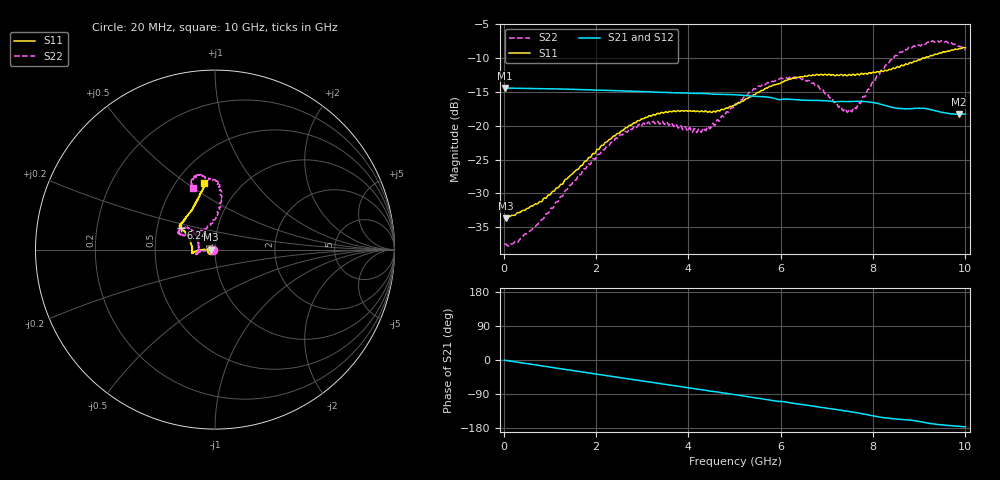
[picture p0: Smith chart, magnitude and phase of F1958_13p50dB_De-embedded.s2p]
! Integrated Device Technology
! Corporate Headquarters
! 6024 Silver Creek Valley Road
! San Jose, CA 95138  USA
! Phone:  1-408-284-8200
! Toll Free:  1-800-223-1366
! Webpage:  http://www.idt.com/
! Timing and RF Division
! 515 Groton Road, Suite 102
! Westford, MA 01886-6024
! Device:  F1958
! Description: 7-bit 0.25 dB Digital Step Attenuator
! Frequency:  0.001 -  6.000 GHz
! Package:  4x4 mm Thin QFN Plastic Package: 24 pin
! Ports:  2 RF, 12 DC
!  Pin  1  = D0
!  Pin  2  = VDD
!  Pin  3  = VMODE
!  Pin  4  = GND
!  Pin  5  = RF1  =  Port 1
!  Pin  6  = GND
!  Pin  7  = GND
!  Pin  8  = GND
!  Pin  9  = GND
!  Pin 10  = GND
!  Pin 11  = GND
!  Pin 12  = GND
!  Pin 13  = GND
!  Pin 14  = RF2  =  Port 2
!  Pin 15  = GND
!  Pin 16  = LE
!  Pin 17  = CLK
!  Pin 18  = DATA
!  Pin 19  = D6
!  Pin 20  = D5
!  Pin 21  = D4
!  Pin 22  = D3
!  Pin 23  = D2
!  Pin 24  = D1
! State:  54
! Atten State:  13.50 dB
! Voltage:  +3.30 Volts
! Current:  0.258 mA
! Data:  The device was measured on a F1958 evaluation board which has
!  individual transmission lines to the RF pins.  Data was collected
!  using a calibrated network analyzer.  The evaluation board was
!  de-embedded using Automatic Fixture Removal (AFR).
!  The reference plane is the edge of the package pin.
! Misc:
!  Action Tracker AT0419
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# GHz S dB R 50
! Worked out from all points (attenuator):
!   500 points, 20 MHz to 10 GHz, reference 50 ohm
!   highest |S21| = -14.39 dB at 20 MHz (marker M1); lowest = -18.3 dB at 9.86 GHz (marker M2)
!   lowest |S11| = -33.7 dB at 40 MHz (marker M3), VSWR 1.04, Z = 48 - j0.0857 ohm
!   |S11| at or under -10 dB: start of sweep to 9.066 GHz
!   |S22| runs from -37.8 to -7.4 dB; largest |S21 - S12| = 0.00057
!   S11 on the Smith chart (normalised r, x): 20 MHz: 0.96, -0.00; 6.24 GHz: 0.67, +0.17; 10 GHz: 0.68, +0.59
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0.02  -33.63 -177.7  -14.39 -0.5  -14.39 -0.5  -37.57 -176.4
0.04  -33.66 -177.5  -14.40 -0.9  -14.40 -0.9  -37.46 -174.8
0.32  -32.82 178.1  -14.45 -6.1  -14.45 -6.1  -37.08 -178.8
0.72  -31.57 178.8  -14.49 -13.5  -14.48 -13.5  -34.65 -175.4
1.7  -25.83 179.7  -14.64 -31.5  -14.64 -31.5  -26.78 -175.9
2.6  -20.59 -176.7  -14.84 -48.0  -14.82 -48.0  -21.11 -172.5
2.92  -19.24 -174.0  -14.91 -53.8  -14.90 -53.9  -19.82 -169.5
3.36  -18.21 -171.7  -15.04 -61.8  -15.04 -61.9  -19.58 -165.3
4.32  -17.92 -178.0  -15.22 -79.0  -15.23 -79.1  -20.33 166.3
4.64  -17.71 174.1  -15.33 -84.7  -15.34 -84.7  -19.11 153.0
5.02  -16.91 162.6  -15.40 -91.7  -15.41 -91.8  -16.73 141.3
5.54  -15.01 152.1  -15.66 -101.4  -15.67 -101.4  -14.13 142.2
6.24  -13.02 147.9  -16.09 -113.7  -16.11 -113.7  -12.96 153.6
6.68  -12.51 146.0  -16.24 -121.2  -16.25 -121.2  -13.68 155.7
7.32  -12.42 140.4  -16.40 -132.9  -16.40 -132.8  -17.38 135.1
7.5  -12.44 137.3  -16.41 -136.1  -16.41 -136.0  -17.55 117.1
7.68  -12.39 134.3  -16.36 -139.8  -16.36 -139.8  -16.64 99.6
8.34  -11.67 118.5  -17.14 -154.0  -17.14 -154.1  -10.76 82.8
8.68  -11.00 111.7  -17.48 -157.4  -17.48 -157.4  -8.66 87.1
9.26  -9.58 103.6  -17.63 -167.9  -17.63 -168.0  -7.55 99.9
9.86  -8.58 98.9  -18.31 -175.0  -18.34 -174.9  -8.26 109.2
10  -8.45 98.9  -18.25 -176.6  -18.28 -176.5  -8.77 110.1
